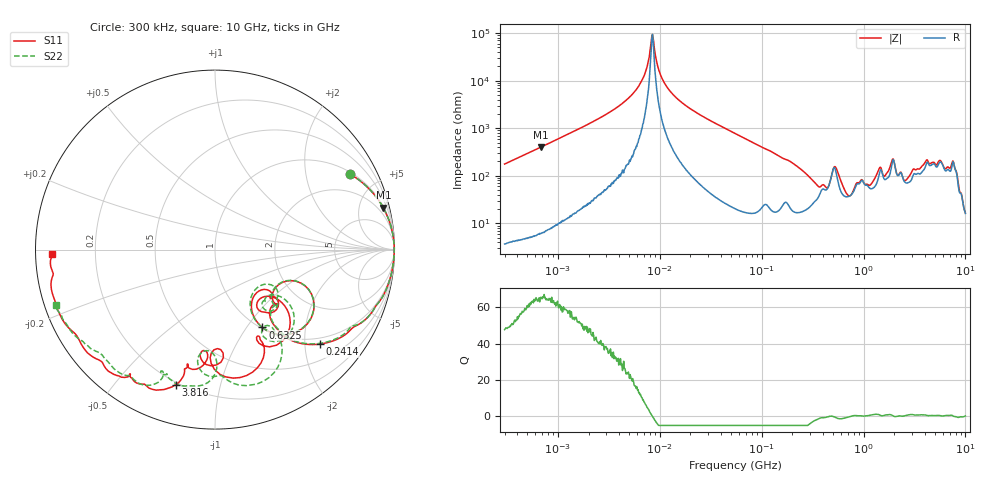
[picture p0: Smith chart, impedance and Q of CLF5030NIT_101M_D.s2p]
! S-Parameter Data Generated by TDK Corporation
! Copyright(C) 2019 TDK Corporation.
! All Rights Reserved.
! TDK P/N: CLF5030NIT-101M-D (Inductor)
! Property: L=100uH at 100kHz
! Size(LxWxT): 5.3x5x2.7mm
! Model Type: s2p (Touchstone File Format Version 1.0)
! Frequency: DC=Yes Start=0.3MHz Stop=10000MHz 802points Log-sweep
! Model Generated on May 10, 2019
! Port Assignments:
!  1 ---@@@--- 2
! Applicable Conditions:
!  Temperature = 25 degC
!  DC Bias Current = 0 A
!  Small Signal Operation
! Terms and conditions regarding TDK Simulation Models
! (1)This simulation model is being provided solely for informational purposes. Please refer to the specifications of the products in terms of detailed characteristics of such products.
! (2)In no event shall TDK Corporation of any of its subsidiaries be liable for any loss or damage arising, directly or indirectly,
!  From any information contained in this simulation model, including, but not limited to loss or damages arising from any inaccuracies, omissions or errors in connection with such information.
! (3)Any and all copyrights on this simulation model are owned by TDK Corporation.
!  Duplication or redistribution of this simulation model without prior written permission from TDK Corporation is prohibited.
! (4)This simulation model is subject to any modification or change without any prior notice.
! (5)Neither TDK Corporation nor any of its subsidiaries shall make any warranty, express or implied,
!  Including but not limited to the correctness, implied warranties of merchantability and fitness for a particular purpose with respect to this simulation models.
! (6)The use of this simulation model shall be deemed to have consented to the terms and conditions hereof.
# Hz S MA R 50
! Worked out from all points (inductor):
!   801 points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, 300 kHz to 10 GHz, reference 50 ohm
!   read as one part in series: L = 93.5 uH near 318.3 kHz
!   highest Q = 65.3 at 680.6 kHz (marker M1), where L = 93.7 uH
!   self-resonance near 8.366 MHz
!   S11 on the Smith chart (normalised r, x): 300 kHz: 1.08, +3.53; 241.4 MHz: 0.85, -2.35; 632.5 MHz: 1.02, -1.19; 3.816 GHz: 0.19, -0.73; 10 GHz: 0.05, -0.01
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300000  0.8625 29.2  0.4881 -59.6  0.4882 -59.6  0.8624 29.2
680647  0.9664 13.9  0.241 -75.2  0.2409 -75.2  0.9663 13.9
1713600  0.9934 5.4  0.09577 -83.4  0.09568 -83.4  0.9934 5.4
5416338  0.9988 0.9  0.01902 -86.4  0.01905 -86.2  0.9989 0.9
7070888  0.9989 0.1  0.007619 -82.5  0.007512 -82.2  0.999 0.1
8484346  0.9988 -0.3  0.001068 1.0  0.001076 -1.0  0.9989 -0.3
9671944  0.9988 -0.7  0.0055 77.7  0.005489 77.4  0.9989 -0.7
1.49005e7  0.9983 -2.0  0.02404 84.7  0.02403 84.7  0.9983 -2.0
5.477226e7  0.9886 -9.5  0.1265 79.0  0.1265 79.0  0.9886 -9.5
2.413764e8  0.7877 -41.9  0.5313 41.6  0.5313 41.6  0.7874 -41.5
3.126428e8  0.607 -51.6  0.6468 23.2  0.6468 23.2  0.6106 -51.0
4.687561e8  0.4361 -23.7  0.5649 -15.2  0.5649 -15.2  0.432 -23.7
5.225392e8  0.6448 -31.4  0.38 -3.4  0.38 -3.4  0.6428 -31.2
6.325141e8  0.5083 -58.6  0.6353 0.5  0.6354 0.5  0.5045 -58.8
1.24442e9  0.4003 -40.6  0.5902 -55.5  0.5904 -55.5  0.4115 -37.7
1.767019e9  0.5922 -63.0  0.3968 -82.2  0.397 -82.3  0.6002 -54.0
2.020878e9  0.6965 -87.7  0.2448 -59.9  0.2448 -59.9  0.7781 -77.0
2.659614e9  0.5661 -95.9  0.3774 -89.8  0.3773 -89.8  0.5722 -96.7
3.816223e9  0.7845 -106.3  0.169 -127.5  0.1693 -127.6  0.7428 -111.2
6.41458e9  0.8927 -136.6  0.08697 -144.3  0.08674 -144.3  0.8619 -137.6
7.875699e9  0.9369 -157.2  0.03175 -130.8  0.03152 -130.3  0.9238 -152.0
1e10  0.9073 -178.6  0.04826 -91.0  0.0478 -91.0  0.936 -160.7
